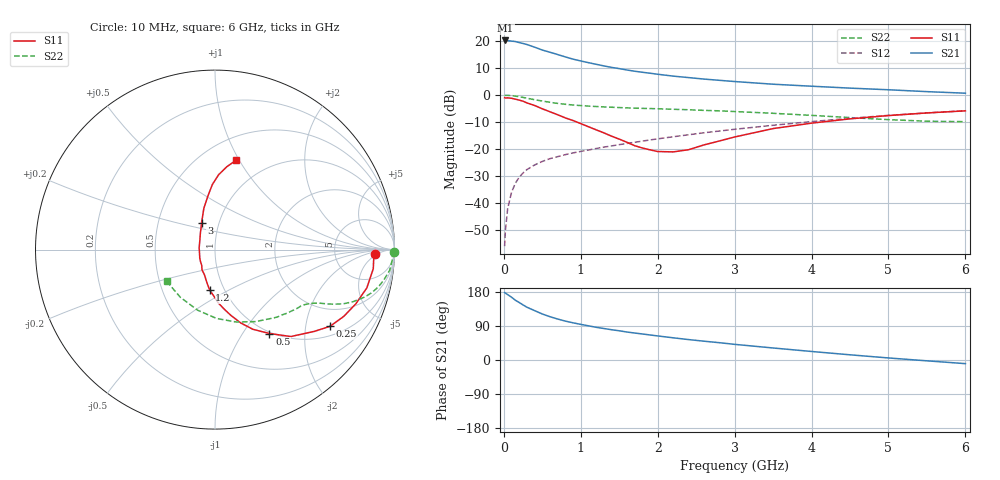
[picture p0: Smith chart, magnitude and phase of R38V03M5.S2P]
! SIEMENS Small Signal Semiconductors
! BFR181
! Si NPN RF Bipolar Junction Transistor in SOT23
! VCE = 8 V  IC = 3.5 mA
! Common Emitter S-Parameters:  May  1996
# GHz  S  MA  R  50
!  f  S11  S21  S12  S22
! GHz  MAG  ANG  MAG  ANG  MAG  ANG  MAG  ANG
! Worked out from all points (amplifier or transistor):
!   36 points, 10 MHz to 6 GHz, reference 50 ohm
!   highest |S21| = 20.2 dB at 20 MHz (marker M1)
!   |S21| within 3 dB of that: start of sweep to 448.4 MHz
!   unconditionally stable (mu >= 1): 1.363 GHz to 3.234 GHz
!   at 250 MHz: K = 0.32, MSG = 24.0 dB, |S12| = -28.8 dB
!   at 1.4 GHz: K = 1.01, MAG = 13.9 dB, |S12| = -18.8 dB
!   at 6 GHz: K = 0.86, MSG = 3.2 dB, |S12| = -5.8 dB
!   S11 on the Smith chart (normalised r, x): 10 MHz: 17, -4; 250 MHz: 1.30, -2.74; 500 MHz: 0.98, -1.33; 1.2 GHz: 0.85, -0.41; 3 GHz: 0.83, +0.25; 6 GHz: 0.72, +0.97
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0.01  0.8924 -1.5  10.19 178.1  0.0016 89.7  0.9949 -0.7
0.02  0.8857 -2.9  10.26 176.5  0.0031 82.8  0.9884 -1.4
0.05  0.8883 -6.9  10.16 172.5  0.008 85.2  0.9889 -3.5
0.1  0.8724 -14.2  9.985 165.7  0.0159 82.7  0.9797 -6.8
0.15  0.8405 -21.1  9.797 157.7  0.0234 77.2  0.9561 -10.2
0.25  0.7703 -33.7  9.021 145.3  0.0362 72.0  0.9066 -15.3
0.3  0.7174 -39.4  8.633 139.3  0.0418 69.5  0.8765 -17.5
0.4  0.6428 -48.9  7.708 130.3  0.0509 65.4  0.8216 -20.7
0.5  0.5574 -57.0  6.819 121.4  0.0592 63.2  0.7761 -22.9
0.6  0.4914 -64.6  6.209 114.2  0.0667 61.6  0.7355 -24.4
0.7  0.4328 -70.7  5.627 108.1  0.0726 60.8  0.702 -25.6
0.8  0.378 -76.3  5.088 102.6  0.0791 60.0  0.6759 -26.4
0.9  0.3383 -80.9  4.628 98.1  0.0852 60.1  0.655 -27.1
1.1  0.2598 -91.3  3.982 90.2  0.0964 60.0  0.6262 -28.5
1.2  0.2276 -97.4  3.715 86.3  0.1027 60.3  0.6146 -29.2
1.6  0.1339 -122.8  2.915 73.8  0.1275 60.6  0.5805 -32.2
2.2  0.0889 173.4  2.247 58.6  0.1694 60.1  0.5464 -38.8
3  0.1678 116.5  1.783 41.3  0.2329 56.7  0.4963 -50.5
3.5  0.2401 104.9  1.59 31.7  0.2765 53.3  0.4604 -60.6
4.5  0.3632 92.3  1.346 13.7  0.3722 44.0  0.3837 -88.7
5.5  0.4673 81.8  1.159 -2.2  0.4694 31.9  0.3285 -125.9
6  0.5112 76.7  1.084 -9.6  0.5141 25.0  0.3223 -146.8
